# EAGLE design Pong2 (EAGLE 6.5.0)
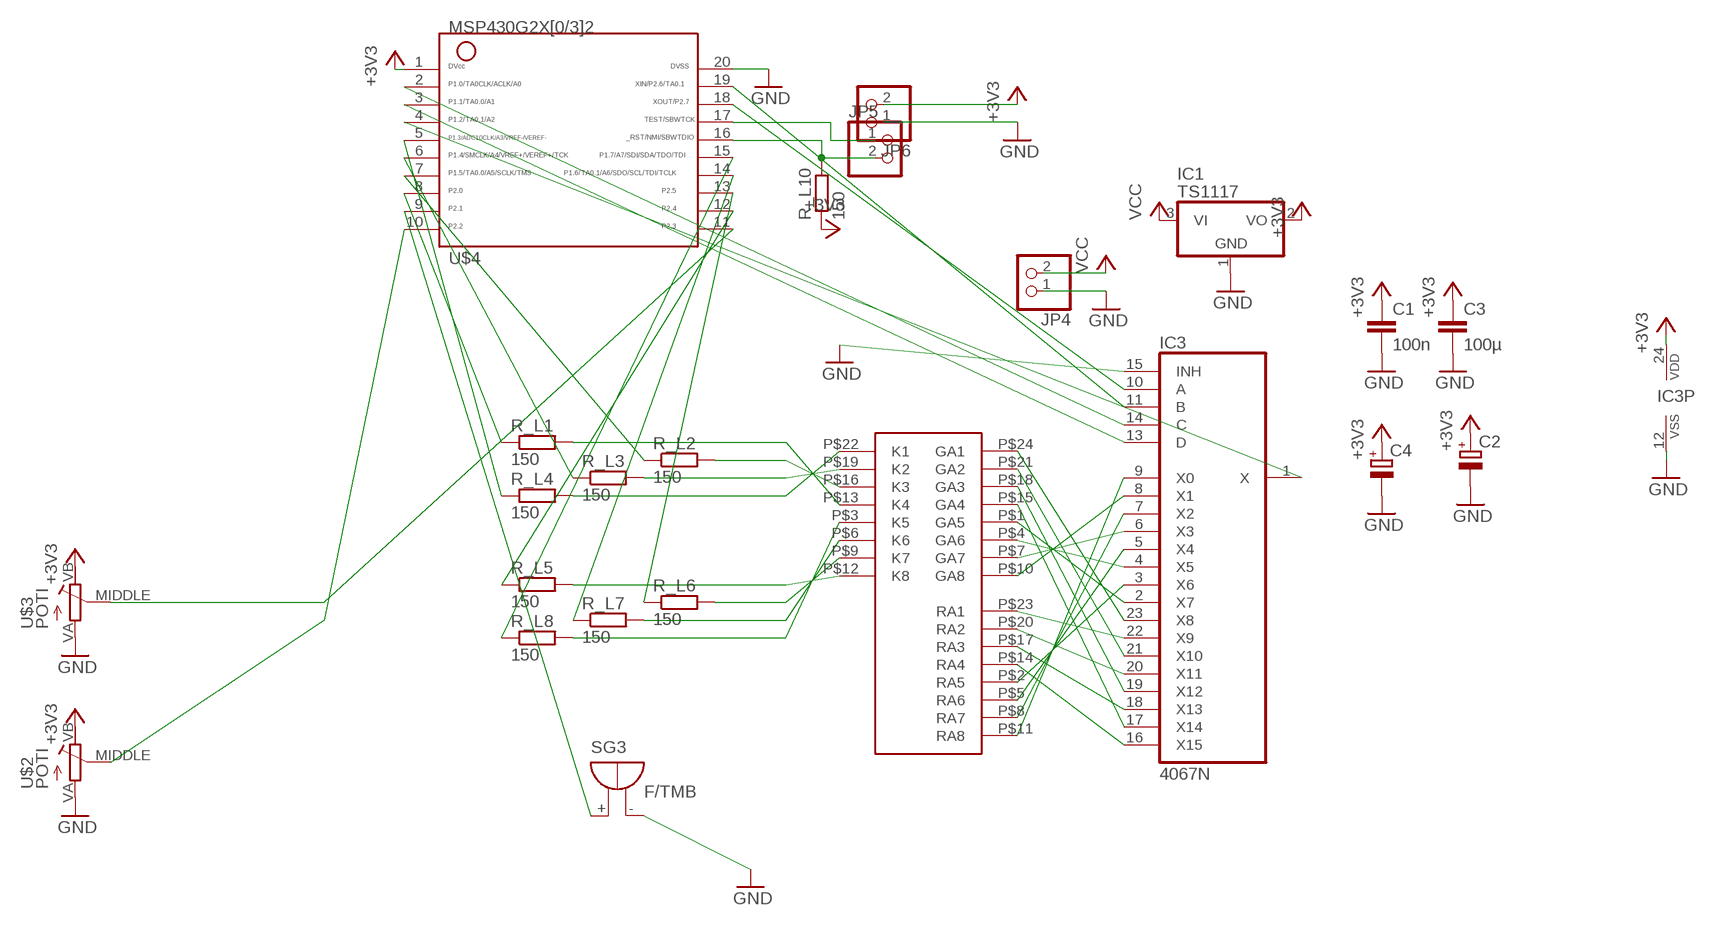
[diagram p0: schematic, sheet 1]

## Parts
C1  100n  C-EUC0603  [C0603]
C2  CPOL-EUE2.5-5  [E2,5-5]
C3  100µ  C-EUC0603  [C0603]
C4  CPOL-EUE2.5-5  [E2,5-5]
IC1  TS1117  [SOT223]
IC3  4067N  [DIL24-6]
JP4  PINHD-1X2  [1X02]
JP5  PINHD-1X2  [1X02]
JP6  PINHD-1X2  [1X02]
R_L1  150  R-EU_R0603  [R0603]
R_L2  150  R-EU_R0603  [R0603]
R_L3  150  R-EU_R0603  [R0603]
R_L4  150  R-EU_R0603  [R0603]
R_L5  150  R-EU_R0603  [R0603]
R_L6  150  R-EU_R0603  [R0603]
R_L7  150  R-EU_R0603  [R0603]
R_L8  150  R-EU_R0603  [R0603]
R_L10  150  R-EU_R0603  [R0603]
SG3  F/TMB  [F/TMB]
U$1  LED_MATRIX  [LED_MATRIX]
U$2  POTI  [LINEAR_POTI]
U$3  POTI  [LINEAR_POTI]
U$4  G2X[0/3]2---PW20  [PW20]

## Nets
+3V3: C1.1 C2.+ C3.1 C4.+ IC1.2(VO) IC3.24(VDD) JP6.2 R_L10.1 U$2.VB(E) U$3.VB(E) U$4.1
GND: C1.2 C2.- C3.2 C4.- IC1.1(GND) IC3.12(VSS) IC3.15(INH) JP4.1 JP6.1 SG3.- U$2.VA(A) U$3.VA(A) U$4.20
N$1: JP5.1 U$4.17
N$2: JP5.2 R_L10.2 U$4.16
N$3: IC3.11(B) U$4.19
N$4: IC3.2(X7) U$1.P$1(GA5)
N$5: IC3.3(X6) U$1.P$2(RA5)
N$6: IC3.4(X5) U$1.P$4(GA6)
N$7: IC3.5(X4) U$1.P$5(RA6)
N$8: IC3.6(X3) U$1.P$7(GA7)
N$9: IC3.10(A) U$4.18
N$10: IC3.7(X2) U$1.P$8(RA7)
N$11: IC3.8(X1) U$1.P$10(GA8)
N$12: IC3.9(X0) U$1.P$11(RA8)
N$13: IC3.16(X15) U$1.P$14(RA4)
N$14: IC3.17(X14) U$1.P$15(GA4)
N$15: IC3.18(X13) U$1.P$17(RA3)
N$16: IC3.19(X12) U$1.P$18(GA3)
N$17: IC3.20(X11) U$1.P$20(RA2)
N$18: IC3.21(X10) U$1.P$21(GA2)
N$19: IC3.22(X9) U$1.P$23(RA1)
N$20: IC3.23(X8) U$1.P$24(GA1)
N$21: IC3.14(C) U$4.2
N$22: IC3.13(D) U$4.3
N$23: IC3.1(X) U$4.4
N$24: R_L4.1 U$4.5
N$25: R_L1.2 U$1.P$13(K4)
N$26: R_L2.2 U$1.P$16(K3)
N$27: R_L3.2 U$1.P$19(K2)
N$28: R_L4.2 U$1.P$22(K1)
N$29: R_L5.2 U$1.P$12(K8)
N$30: R_L6.2 U$1.P$9(K7)
N$31: R_L7.2 U$1.P$6(K6)
N$32: R_L8.2 U$1.P$3(K5)
N$33: R_L3.1 U$4.6
N$34: R_L2.1 U$4.7
N$35: R_L1.1 U$4.8
N$36: R_L8.1 U$4.15
N$37: U$3.MIDDLE(S) U$4.11
N$38: R_L7.1 U$4.14
N$39: R_L6.1 U$4.13
N$40: R_L5.1 U$4.12
N$41: SG3.+ U$4.9
N$44: U$2.MIDDLE(S) U$4.10
VCC: IC1.3(VI) JP4.2

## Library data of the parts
C1 C3 = rcl:C-EU: CAPACITOR, European symbol
C2 C4 = rcl:CPOL-EU: POLARIZED CAPACITOR, European symbol
IC1 = welectronic:TS1117
IC3 = 40xx:4067: 16-channel ANALOG MULTIPLEXER
JP4-JP6 = pinhead:PINHD-1X2: PIN HEADER
R_L1-R_L8 R_L10 = rcl:R-EU_: RESISTOR, European symbol
SG3 = buzzer:F/TMB: BUZZER; OC_FARNELL: unknown; OC_NEWARK: unknown
U$1 = thar:LED_MATRIX
U$2 U$3 = thar:POTI
U$4 = TI_MSP430_v16:G2X[0/3]2---PW20: MSP430G2X[0/3]2 MSP430G2x32, MSP430G2x02 TSSOP (PW) 20 Pin Package http://focus.ti.com/docs/prod/folders/print/msp430g2432.html

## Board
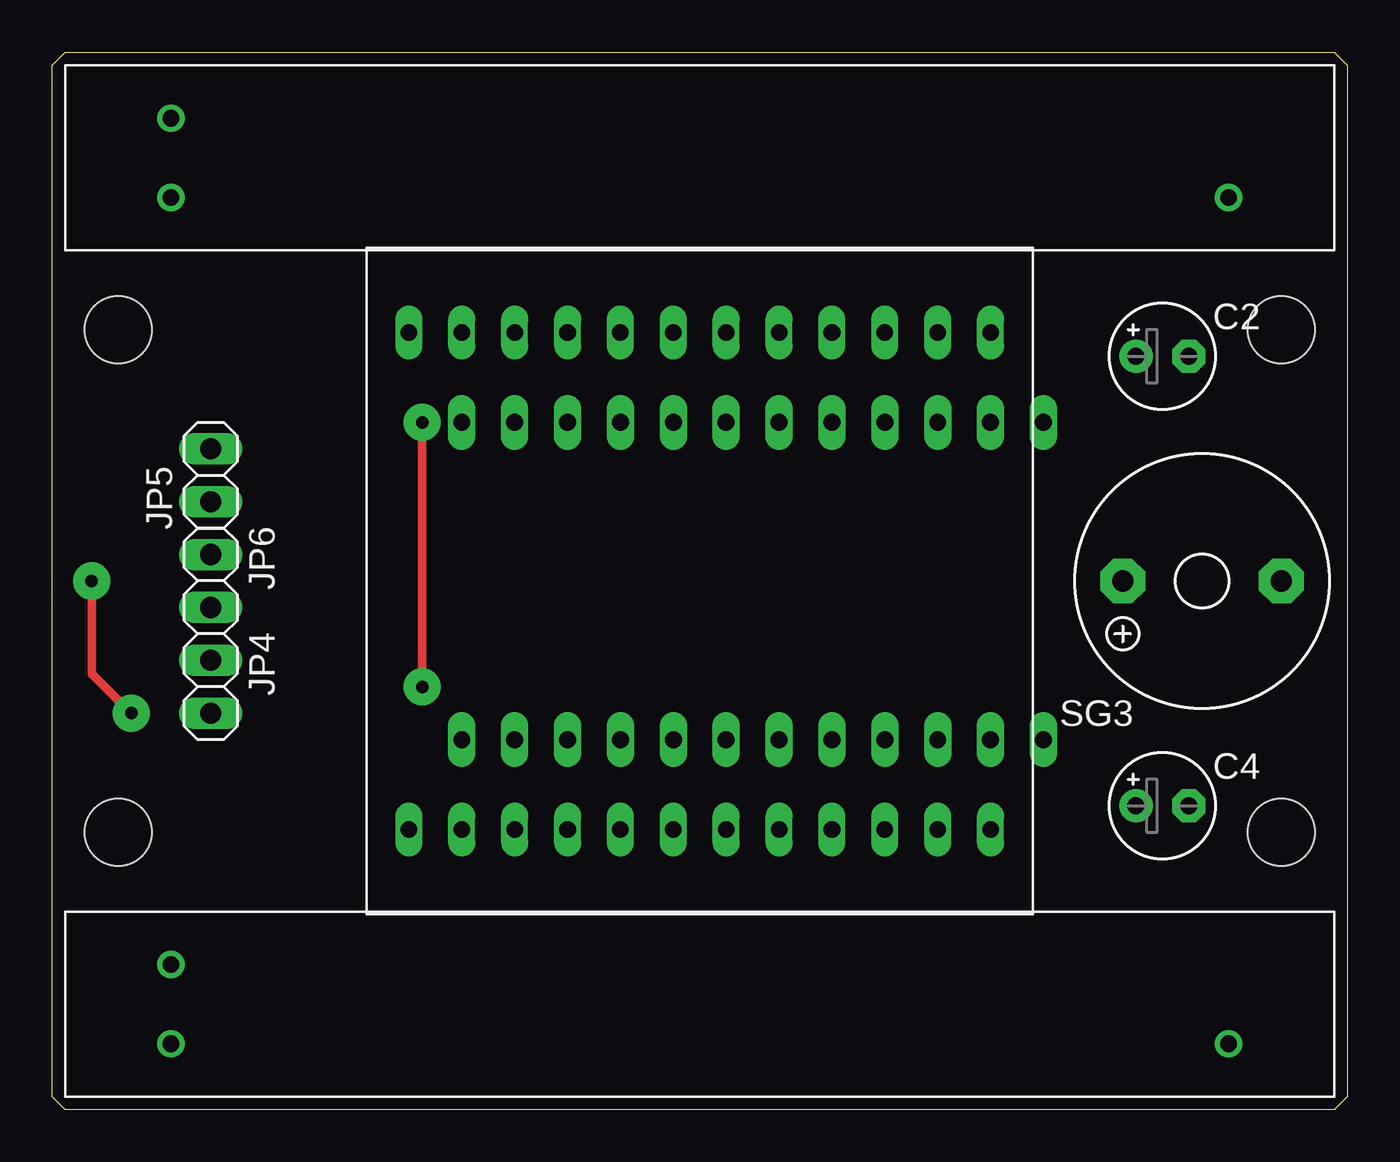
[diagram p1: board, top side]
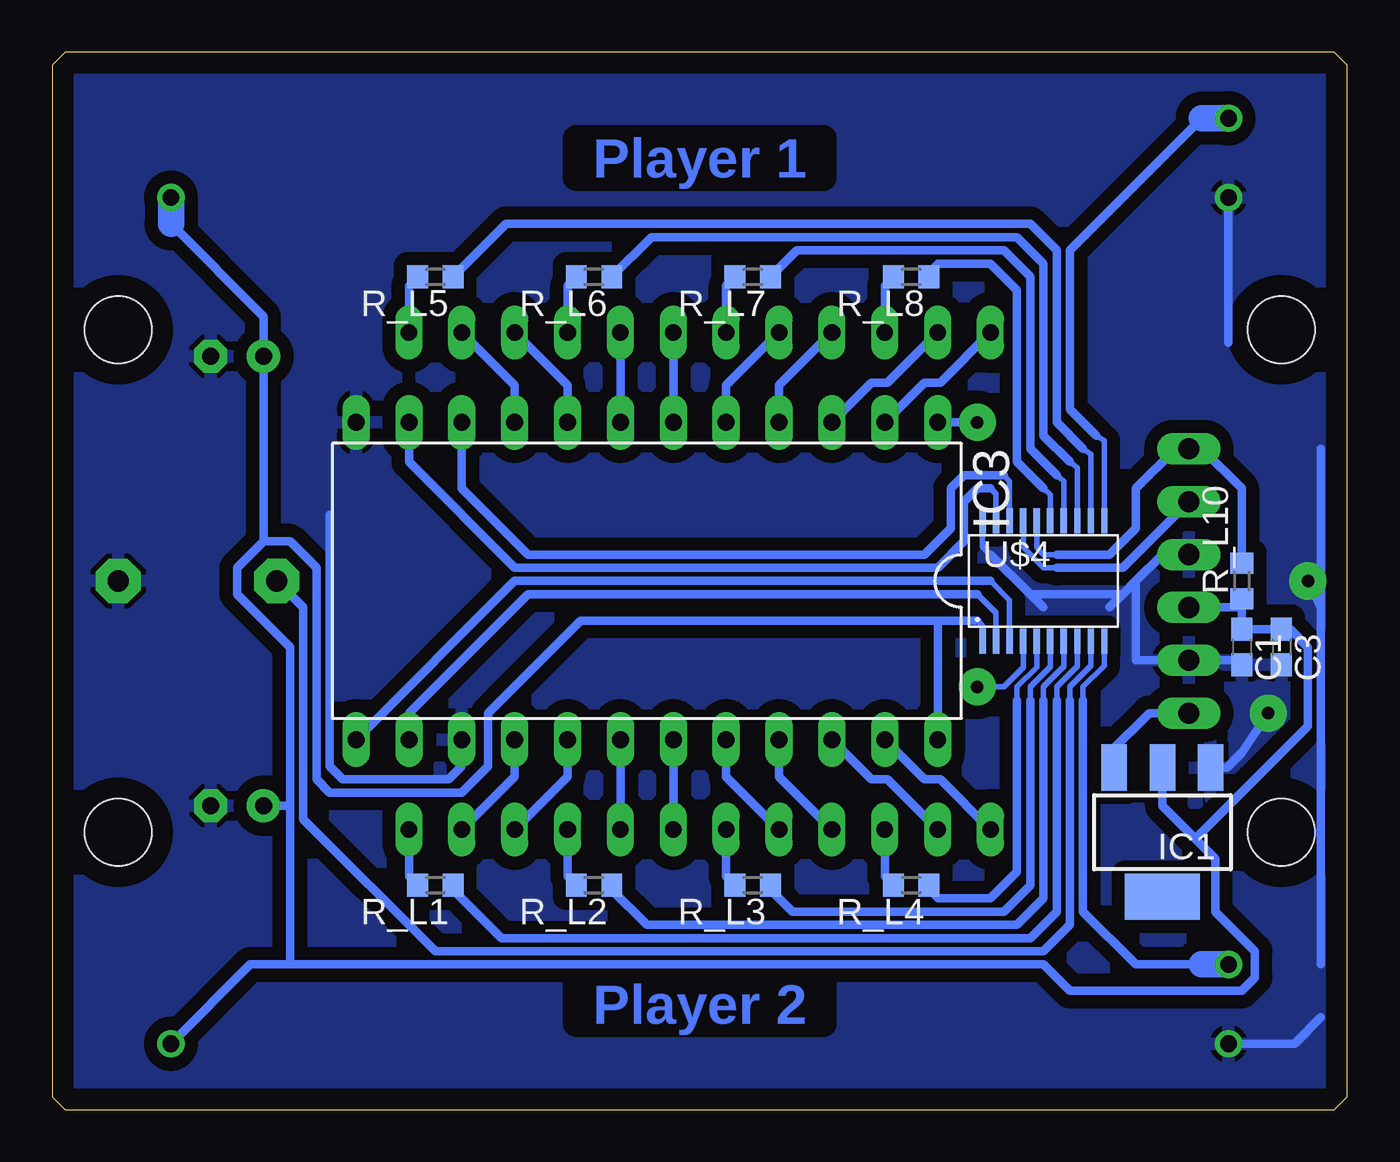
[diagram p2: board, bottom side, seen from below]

Size 62.23 x 50.8 mm. Coordinates in mm from the lower left corner, seen from the top.
Outline: 0.63,50.8 61.6,50.8 62.23,50.16 62.23,0.63 61.6,0 0.63,0 0,0.63 0,50.16 0.63,50.8
Copper layers (1*16): Top 0.035mm / dielectric 1.5mm / Bottom 0.035mm
Design rules "default": minimum track width 10mil, minimum drill 24mil, track to track 8mil, track to pad 8mil, pad to pad 8mil, via to via 8mil, smd to smd 8mil, copper to edge 40mil, drill to drill 8mil, minimum pad ring 10mil, minimum via ring 8mil, stop-mask expansion 4mil, vias tented up to drill 0mil, thermal gap 10mil
Holes 3.2 mm at 59.05,37.47 59.05,13.34 3.18,13.34 3.18,37.47

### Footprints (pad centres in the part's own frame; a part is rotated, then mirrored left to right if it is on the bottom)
C0603 = smd 1.1 x 1: 1 -0.85,0; 2 0.85,0
E2,5-5 = drill 0.813 pad 1.6: + -1.27,0 | drill 0.813 pad 1.6 octagon: - 1.27,0
SOT223 = smd 1.219 x 2.235: 1 -2.311,-3.099; 2 0,-3.099; 3 2.311,-3.099 | smd 3.6 x 2.2: 4 0,3.099
DIL24-6 = drill 0.813 long: 1 -13.97,-7.62; 2 -11.43,-7.62; 3 -8.89,-7.62; 4 -6.35,-7.62; 5 -3.81,-7.62; 6 -1.27,-7.62; 7 1.27,-7.62; 8 3.81,-7.62; 9 6.35,-7.62; 10 8.89,-7.62; 11 11.43,-7.62; 12 13.97,-7.62; 13 13.97,7.62; 14 11.43,7.62; 15 8.89,7.62; 16 6.35,7.62; 17 3.81,7.62; 18 1.27,7.62; 19 -1.27,7.62; 20 -3.81,7.62; 21 -6.35,7.62; 22 -8.89,7.62; 23 -11.43,7.62; 24 -13.97,7.62
1X02 = drill 1.016 long: 1 -1.27,0; 2 1.27,0
R0603 = smd 1 x 1.1: 1 -0.85,0; 2 0.85,0
F/TMB = drill 1.016 pad 2.159 octagon: + 3.81,0; - -3.81,0
LED_MATRIX = drill 0.8 long: P$1 -13.97,11.938; P$2 -11.43,11.938; P$3 -8.89,11.938; P$4 -6.35,11.938; P$5 -3.81,11.938; P$6 -1.27,11.938; P$7 1.27,11.938; P$8 3.81,11.938; P$9 6.35,11.938; P$10 8.89,11.938; P$11 11.43,11.938; P$12 13.97,11.938; P$13 13.97,-11.938; P$14 11.43,-11.938; P$15 8.89,-11.938; P$16 6.35,-11.938; P$17 3.81,-11.938; P$18 1.27,-11.938; P$19 -1.27,-11.938; P$20 -3.81,-11.938; P$21 -6.35,-11.938; P$22 -8.89,-11.938; P$23 -11.43,-11.938; P$24 -13.97,-11.938
LINEAR_POTI = drill 0.8: MIDDLE -7.62,6.35; VA -7.62,2.54; VB 43.18,2.54
PW20 = smd 0.3 x 1.2: 1 -2.925,-2.9; 2 -2.275,-2.9; 3 -1.625,-2.9; 4 -0.975,-2.9; 5 -0.325,-2.9; 6 0.325,-2.9; 7 0.975,-2.9; 8 1.625,-2.9; 9 2.275,-2.9; 10 2.925,-2.9; 11 2.925,2.9; 12 2.275,2.9; 13 1.625,2.9; 14 0.975,2.9; 15 0.325,2.9; 16 -0.325,2.9; 17 -0.975,2.9; 18 -1.625,2.9; 19 -2.275,2.9; 20 -2.925,2.9

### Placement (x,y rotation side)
C1  5.08,22.23 270 bottom
C2  53.34,36.2 0 top
C3  3.18,22.23 270 bottom
C4  53.34,14.61 0 top
IC1  8.89,13.34 180 bottom
IC3  33.66,25.4 180 bottom
JP4  7.62,20.32 270 top
JP5  7.62,30.48 90 top
JP6  7.62,25.4 270 top
R_L1  43.82,10.8 180 bottom
R_L2  36.2,10.8 180 bottom
R_L3  28.58,10.8 180 bottom
R_L4  20.95,10.8 180 bottom
R_L5  43.82,40.01 180 bottom
R_L6  36.2,40.01 180 bottom
R_L7  28.58,40.01 180 bottom
R_L8  20.95,40.01 180 bottom
R_L10  5.08,25.4 90 bottom
SG3  55.24,25.4 180 top
U$1  31.12,25.4 0 top
U$2  13.34,0.63 0 top
U$3  13.34,41.27 0 top
U$4  14.6,25.4 0 bottom

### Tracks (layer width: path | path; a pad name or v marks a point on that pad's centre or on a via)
+3V3
  Bottom 0.254: JP6.2 5.29,24.13 | 5.29,24.13 5.08,24.13 R_L10.1 5.29,24.13 | U$4.1 17.53,23.25 17.78,23.5
  Bottom 0.406: JP6.2 5.08,24.13 C1.1 | 50.8,14.61 50.8,22.23 53.34,24.77 53.34,26.04 52.07,27.3 | 52.07,27.3 C2.+ 52.07,38.1 56.51,42.55 | C3.1 C1.1 | 17.78,23.5 19.69,23.5 | 19.69,23.5 36.83,23.5 41.27,19.05 41.27,16.51 42.55,15.24 48.9,15.24 49.53,15.88 49.53,26.04 50.8,27.3 52.07,27.3 | U$2.VB 52.71,6.99 51.43,6.99 50.8,6.99 | 50.8,6.99 50.8,14.61 | 50.8,14.61 C4.+ | 50.8,6.99 14.6,6.99 13.34,5.72 5.08,5.72 4.45,6.35 4.45,7.62 6.35,9.52 6.35,12.07 7.3,13.02 | 7.3,13.02 8.89,14.61 IC1.2 | C1.1 2.75,23.07 1.91,22.23 1.91,18.41 7.3,13.02 | IC3.24 19.69,23.5
  Bottom 1.27: U$3.VB 56.51,42.55
GND  (via drill 0.6 pad 1.78)
  Top 0.406: v1.91,25.4 1.91,20.96 v3.81,19.05
  Bottom 0.254: 5.71,21.59 5.29,21.59 | 5.29,21.59 C1.2 | 5.29,21.59 5.08,21.59 | U$4.20 17.53,27.05 17.15,26.67
  Bottom 0.406: U$3.VA 5.71,36.83 | 1.27,31.75 1.27,24.13 | C1.2 5.08,21.59 5.71,21.59 JP4.1 10.16,21.59 10.16,25.4 | 1.27,6.99 1.27,24.13 | 1.27,24.13 v1.91,25.4 | U$2.VA 2.54,3.17 1.27,4.45 | IC1.1 5.79,16.43 5.08,17.14 v3.81,19.05 | JP6.1 8.89,26.67 10.16,25.4 | 10.16,25.4 10.79,24.77 | 11.43,24.13 10.79,24.77 | 10.79,24.77 15.24,24.77 | 15.24,24.77 17.15,26.67 | 15.24,24.77 14.6,24.13 | IC3.15 42.55,16.51 43.18,15.88 48.26,15.88 48.9,16.51 48.9,28.57
  pour Bottom (isolate 0.635): 0.63,0.63 0.63,50.16 61.6,50.16 61.6,0.63
N$1
  Bottom 0.254: U$4.17 15.58,27.01 14.6,26.04 13.97,26.04
  Bottom 0.406: JP5.1 10.79,26.04 13.97,26.04
N$2
  Bottom 0.254: U$4.16 14.93,27 14.6,26.67 13.97,26.67 | 5.08,26.67 R_L10.2
  Bottom 0.406: 5.08,26.67 5.08,29.84 6.98,31.75 JP5.2 8.25,31.75 10.16,29.84 10.16,27.94 11.43,26.67 13.97,26.67
N$3
  Bottom 0.254: U$4.19 16.88,29.58 17.15,29.84
  Bottom 0.406: IC3.11 45.09,31.12 40.01,26.04 19.69,26.04 18.41,27.3 18.41,29.21 17.78,29.84 17.15,29.84
N$4
  Bottom 0.406: IC3.2 20.32,34.93 19.56,34.93 U$1.P$1
N$5
  Bottom 0.406: IC3.3 22.86,34.93 22.1,34.93 U$1.P$2
N$6
  Bottom 0.406: IC3.4 27.3,34.8 U$1.P$4
N$7
  Bottom 0.406: IC3.5 29.84,34.8 U$1.P$5
N$8
  Bottom 0.406: IC3.6 U$1.P$7
N$9
  Bottom 0.254: U$4.18 16.23,30.2 16.51,30.48
  Bottom 0.406: IC3.10 42.55,29.84 39.37,26.67 20.32,26.67 19.05,27.94 19.05,29.84 18.41,30.48 16.51,30.48
N$10
  Bottom 0.406: IC3.7 U$1.P$8
N$11
  Bottom 0.406: IC3.8 37.46,34.8 U$1.P$10
N$12
  Bottom 0.406: IC3.9 40.01,34.8 U$1.P$11
N$13
  Bottom 0.406: IC3.16 40.01,16 U$1.P$14
N$14
  Bottom 0.406: IC3.17 37.46,16 U$1.P$15
N$15
  Bottom 0.406: IC3.18 U$1.P$17
N$16
  Bottom 0.406: IC3.19 U$1.P$18
N$17
  Bottom 0.406: IC3.20 29.84,16 U$1.P$20
N$18
  Bottom 0.406: IC3.21 27.3,16 U$1.P$21
N$19
  Bottom 0.406: IC3.22 22.86,15.88 22.1,15.88 U$1.P$23
N$20
  Bottom 0.406: IC3.23 20.32,15.88 19.56,15.88 U$1.P$24
N$21
  Bottom 0.254: U$4.2 16.88,23.87 17.78,24.77
  Bottom 0.406: IC3.14 45.09,19.05 39.37,24.77 17.78,24.77
N$22
  Bottom 0.254: U$4.3 16.23,24.48 17.15,25.4
  Bottom 0.406: IC3.13 40.01,25.4 17.15,25.4
N$23  (via drill 0.6 pad 1.78)
  Top 0.406: v17.78,33.02 v17.78,20.32
  Bottom 0.254: U$4.4 15.58,21.25 16.51,20.32 17.15,20.32
  Bottom 0.406: IC3.1 v17.78,33.02 | v17.78,20.32 17.15,20.32
N$24
  Bottom 0.254: U$4.5 14.93,21.27 15.88,20.32 15.88,19.69
  Bottom 0.406: R_L4.1 20.1,10.58 19.69,10.16 17.15,10.16 15.88,11.43 15.88,19.69
N$25
  Bottom 0.406: R_L1.2 45.09,11.21 U$1.P$13
N$26
  Bottom 0.406: R_L2.2 37.46,11.21 U$1.P$16
N$27
  Bottom 0.406: U$1.P$19 29.84,11.21 R_L3.2
N$28
  Bottom 0.406: R_L4.2 22.23,11.21 U$1.P$22
N$29
  Bottom 0.406: R_L5.2 45.09,39.59 U$1.P$12
N$30
  Bottom 0.406: R_L6.2 37.46,39.59 U$1.P$9
N$31
  Bottom 0.406: R_L7.2 29.84,39.59 U$1.P$6
N$32
  Bottom 0.406: R_L8.2 22.23,39.59 U$1.P$3
N$33
  Bottom 0.254: U$4.6 14.28,21.28 15.24,20.32 15.24,19.69
  Bottom 0.406: R_L3.1 27.94,10.8 26.67,9.52 16.51,9.52 15.24,10.8 15.24,19.69
N$34
  Bottom 0.254: U$4.7 13.63,21.3 14.6,20.32 14.6,19.69
  Bottom 0.406: R_L2.1 35.34,10.58 33.66,8.89 15.88,8.89 14.6,10.16 14.6,19.69
N$35
  Bottom 0.254: U$4.8 12.98,21.31 13.97,20.32 13.97,19.69
  Bottom 0.406: R_L1.1 42.96,10.58 40.64,8.25 15.24,8.25 13.97,9.52 13.97,19.69
N$36
  Bottom 0.254: U$4.15 14.28,29.54 14.6,29.84
  Bottom 0.406: R_L8.1 20.1,40.22 19.69,40.64 17.15,40.64 15.88,39.37 15.88,31.12 14.6,29.84
N$37
  Bottom 0.254: U$4.11 11.68,32.13 12.06,32.38
  Bottom 0.406: 6.98,47.62 13.34,41.27 13.34,33.66 12.06,32.38
  Bottom 1.27: U$3.MIDDLE 6.98,47.62
N$38
  Bottom 0.254: U$4.14 13.63,30.19 13.97,30.48
  Bottom 0.406: R_L7.1 26.45,41.27 16.51,41.27 15.24,40.01 15.24,31.75 13.97,30.48
N$39
  Bottom 0.254: U$4.13 12.98,30.84 13.34,31.12
  Bottom 0.406: R_L6.1 33.44,41.91 15.88,41.91 14.6,40.64 14.6,32.38 13.34,31.12
N$40
  Bottom 0.254: U$4.12 12.33,31.48 12.7,31.75
  Bottom 0.406: R_L5.1 40.42,42.55 15.24,42.55 13.97,41.27 13.97,33.02 12.7,31.75
N$41
  Bottom 0.254: U$4.9 12.33,21.32 13.34,20.32 13.34,19.69
  Bottom 0.406: 13.34,19.69 13.34,8.89 14.6,7.62 43.82,7.62 50.16,13.97 50.16,24.13 SG3.+
N$44
  Bottom 0.254: U$4.10 11.68,21.34 12.7,20.32 12.7,19.69
  Bottom 0.406: 12.7,19.69 12.7,9.52 10.16,6.99 6.98,6.99
  Bottom 1.27: U$2.MIDDLE 6.98,6.99
VCC
  Bottom 0.406: JP4.2 9.52,19.05 11.43,17.14 11.43,16.66 IC1.3

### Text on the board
Bottom: Player 1 | Player 2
